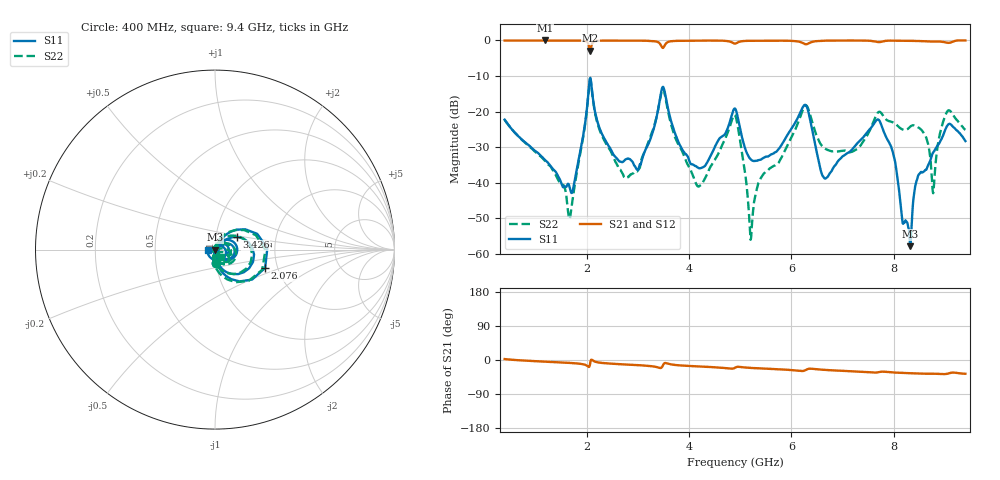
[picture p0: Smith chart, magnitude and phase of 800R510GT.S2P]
!  American Technical Ceramics  Date:  6/19/09
!  One Norden Lane
!  Huntington Station,  NY.  11746-2102
!  Tel:  (631) 622-4700  Fax:  (631) 622-4748
!  Part Number  800R510GT
!  Description: Ultra-low ESR, NPO  Mounting Orientation: Horizontal
!  Application: High RF power Filters, Combiners, Matching networks,
!  Antenna, DC block, Bypass and Couplers
# GHZ S DB R 50
! Freq  |S11|  S11 Ph  |S21|  S21 Ph  |S12|  S12 Ph  |S22|  S22 Ph
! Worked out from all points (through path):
!   801 points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, 400 MHz to 9.4 GHz, reference 50 ohm
!   highest |S21| = -0.01 dB at 1.188 GHz (marker M1); lowest = -2.9 dB at 2.076 GHz (marker M2)
!   group delay of S21, straight-line fit = 11.5 ps
!   lowest |S11| = -57.9 dB at 8.32 GHz (marker M3), VSWR 1.00, Z = 50.1 - j0.099 ohm
!   |S11| at or under -10 dB: start of sweep to end of sweep
!   |S22| runs from -56.1 to -10.9 dB; largest |S21 - S12| = 0.0054
!   S11 on the Smith chart (normalised r, x): 400 MHz: 1.00, -0.15; 2.076 GHz: 1.72, -0.39; 3.426 GHz: 1.26, +0.18; 9.4 GHz: 0.93, -0.00
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0.4  -22.28 -86.1  -0.03 2.5  -0.06 2.6  -22.28 -86.6
1.188  -33.60 -83.8  -0.01 -4.4  -0.04 -4.3  -33.85 -97.9
1.671  -41.37 -22.7  -0.03 -7.7  -0.06 -7.6  -50.31 158.7
1.908  -29.02 58.5  -0.08 -10.6  -0.10 -10.5  -29.42 75.6
2.076  -10.53 -20.1  -2.90 -4.6  -2.92 -4.5  -10.87 -23.1
2.763  -33.48 -36.7  -0.07 -11.7  -0.10 -11.6  -38.62 -124.6
3.033  -35.38 10.2  -0.03 -13.7  -0.05 -13.6  -36.00 156.7
3.404  -19.01 36.8  -0.54 -20.0  -0.56 -19.9  -19.02 43.0
3.426  -17.14 30.3  -0.80 -20.8  -0.82 -20.7  -17.27 34.3
4.191  -35.95 -16.4  -0.07 -16.9  -0.08 -16.8  -41.12 145.9
4.9  -19.17 -11.4  -0.90 -20.4  -0.91 -20.2  -21.06 -18.3
5.215  -33.57 -18.2  -0.10 -20.9  -0.11 -20.8  -55.52 3.3
5.429  -33.32 17.1  -0.09 -22.4  -0.10 -22.3  -38.16 42.9
6.25  -18.25 7.8  -0.93 -28.3  -0.94 -28.1  -18.70 -5.5
6.408  -25.13 -54.4  -0.41 -23.2  -0.40 -23.0  -22.91 -70.7
6.666  -38.87 2.7  -0.06 -26.2  -0.06 -26.0  -30.52 -65.3
7.668  -22.38 7.2  -0.40 -33.0  -0.38 -32.8  -20.83 -32.2
7.904  -28.60 -61.5  -0.06 -32.0  -0.05 -31.8  -22.69 -69.2
8.32  -57.89 -50.8  -0.11 -34.8  -0.10 -34.6  -24.31 -67.4
8.77  -31.58 67.6  -0.30 -36.2  -0.28 -36.0  -43.00 -48.0
9.04  -24.10 -11.5  -0.65 -36.5  -0.63 -36.2  -20.10 -19.8
9.4  -28.32 -179.0  -0.01 -36.3  -0.01 -36.0  -25.16 -49.1
